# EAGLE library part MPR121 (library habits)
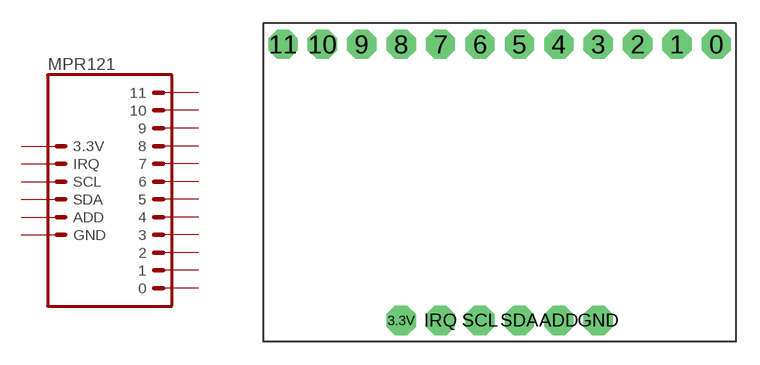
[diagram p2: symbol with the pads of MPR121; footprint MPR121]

Designator prefix -

## MPR121  [MPR121]
0  0  pas
1  1  pas
2  2  pas
3  3  pas
3.3V  3.3V  pas
4  4  pas
5  5  pas
6  6  pas
7  7  pas
8  8  pas
9  9  pas
10  10  pas
11  11  pas
ADD  ADD  pas
GND  GND  pas
IRQ  IRQ  pas
SCL  SCL  pas
SDA  SDA  pas

## Footprint MPR121 (pad centres in mm)
Plated Through Hole - 2x12 Specifications: Pin count:24 Pin pitch:0.1" Example device(s): CONN_12x2
drill 1.016 pad 1.88 octagon: 0 13.97,8.9; 1 11.43,8.9; 2 8.89,8.9; 3 6.35,8.9; 3.3V -6.35,-8.9; 4 3.81,8.9; 5 1.27,8.9; 6 -1.27,8.9; 7 -3.81,8.9; 8 -6.35,8.9; 9 -8.89,8.9; 10 -11.43,8.9; 11 -13.97,8.9; ADD 3.81,-8.9; GND 6.35,-8.9; IRQ -3.81,-8.9; SCL -1.27,-8.9; SDA 1.27,-8.9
